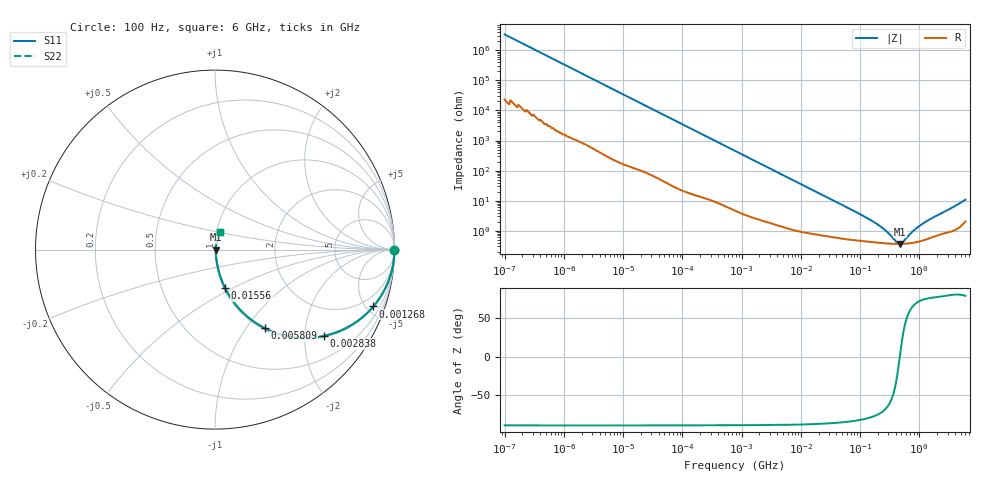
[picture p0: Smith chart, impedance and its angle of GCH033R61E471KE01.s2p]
!Murata Part Number: GCH033R61E471KE01
!These Parameters are Measured in Series Mode Connection
!Data Generated on Jun 19, 2026
!  o--ll--o
!Port1  Port2
!  o------o
!Operation Temp=25[degC], DC Bias Voltage=0[V]
!Freq. Start=100[Hz] Stop=6[GHz] 401[Steps]
# Hz S RI R 50
!Freq.(Hz) S11(Real) S11(Imag) S21(Real) S21(Imag) S12(Real) S12(Imag) S22(Real) S22(Imag)
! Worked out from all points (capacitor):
!   401 points, 100 Hz to 6 GHz, reference 50 ohm
!   read as one part in series: C = 470 pF near 109 Hz
!   lowest |Z| = 364 mohm at 467.5 MHz (marker M1)
!   series resonance near 468.9 MHz, so ESL is about 250 pH
!   S11 on the Smith chart (normalised r, x): 100 Hz: open; 1.268 MHz: 1.06, -5.54; 2.838 MHz: 1.04, -2.49; 5.809 MHz: 1.02, -1.22; 15.56 MHz: 1.02, -0.46; 6 GHz: 1.04, +0.21
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100  1 -2.96e-05  2e-07 2.96e-05  2e-07 2.96e-05  1 -2.96e-05
350  1 -0.000103  6e-07 0.000103  6e-07 0.000103  1 -0.000103
2008  1 -0.000587  3.2e-06 0.000587  3.2e-06 0.000587  1 -0.000587
40335  0.9998 -0.0117  0.000208 0.0117  0.000208 0.0117  0.9998 -0.0117
241822  0.9946 -0.0691  0.00538 0.0691  0.00538 0.0691  0.9946 -0.0691
774597  0.9515 -0.2099  0.0485 0.2099  0.0485 0.2099  0.9515 -0.2099
1267578  0.882 -0.317  0.118 0.317  0.118 0.317  0.882 -0.317
1896632  0.7721 -0.4131  0.2279 0.4131  0.2279 0.4131  0.7721 -0.4131
2837864  0.606 -0.4812  0.394 0.4812  0.394 0.4812  0.606 -0.4812
5809218  0.2759 -0.4373  0.7241 0.4373  0.7241 0.4373  0.2759 -0.4373
9090158  0.1391 -0.3341  0.8609 0.3341  0.8609 0.3341  0.1391 -0.3341
1.555665e7  0.0568 -0.2151  0.9432 0.2151  0.9432 0.2151  0.0568 -0.2151
3.983537e7  0.0138 -0.0887  0.9862 0.0887  0.9862 0.0887  0.0138 -0.0887
1.334425e8  0.00498 -0.0254  0.995 0.0254  0.995 0.0254  0.00498 -0.0254
2.183701e8  0.0041 -0.0135  0.9959 0.0135  0.9959 0.0135  0.0041 -0.0135
3.124326e8  0.00375 -0.00676  0.9963 0.00676  0.9963 0.00676  0.00375 -0.00676
4.087225e8  0.00363 -0.00225  0.9964 0.00225  0.9964 0.00225  0.00363 -0.00225
4.674818e8  0.00363 -4.92e-05  0.9964 4.92e-05  0.9964 4.92e-05  0.00363 -4.92e-05
5.346885e8  0.00366 0.00215  0.9963 -0.00215  0.9963 -0.00215  0.00366 0.00215
8.000355e8  0.00406 0.00914  0.9959 -0.00914  0.9959 -0.00914  0.00406 0.00914
1.144649e9  0.00495 0.0164  0.995 -0.0164  0.995 -0.0164  0.00495 0.0164
6e9  0.0304 0.1007  0.9696 -0.1007  0.9696 -0.1007  0.0304 0.1007
